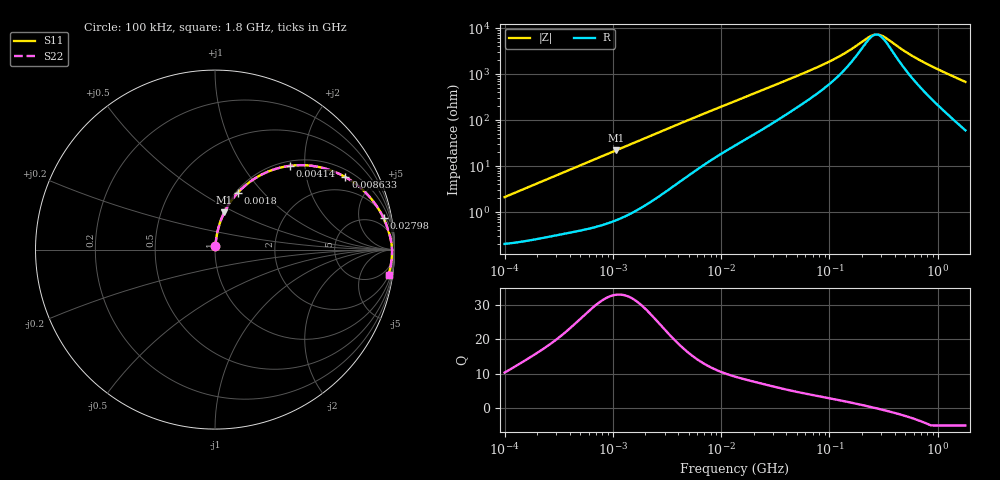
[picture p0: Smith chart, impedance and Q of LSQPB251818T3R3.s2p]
! LSQPB251818T3R3  S-PARAMETER MODEL  ( General Type )
! Model Generated by TAIYO YUDEN Corporation (http://www.ty-top.com)
! Version 2.0
! TAIYO YUDEN Control No. 100810NG19SB-FKC
! Copyright(c) 2009 TAIYO YUDEN CO.,LTD. All Rights Reserved.
! Product Description (link to TY-COMPAS)
! https://ds.yuden.co.jp/TYCOMPAS/or/detail?pn=LSQPB251818T3R3M&u=M
! Products Name : Inductors
! Characteristics :
!  Inductance : 3.3 uH , SRF(min) : 150 MHz , DC Resistance(max) : 0.2275 Ohm
!  Rated Current : Saturation :1450 mA , Temp Rise : 860 mA (40 degC)
!  Case Size : 2.5 x 1.8 / 0.098 x 0.071 [mm/inch] , Thickness : 1.8 / 0.071 [mm/inch]
!  (Conditions: Temperature = 25 degC , DC Bias Current/Voltage = 0A / 0V)
! External Node Assignments :
!  1  o---GGG---o  2
! GND o---------o GND
! Frequency Range : 0.1MHz  -  1800MHz  [ 402 STEP ]
# MHz S RI R 50
! Freq[MHz].  S11 Real  S11 Imag  S21 Real  S21 Imag  S12 Real  S12 Imag  S22 Real  S22 Imag
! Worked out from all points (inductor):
!   401 points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, 100 kHz to 1.8 GHz, reference 50 ohm
!   read as one part in series: L = 3.35 uH near 105 kHz
!   highest Q = 33 at 1.076 MHz (marker M1), where L = 3.26 uH
!   self-resonance near 270.2 MHz
!   S11 on the Smith chart (normalised r, x): 100 kHz: 1.00, +0.04; 1.8 MHz: 1.02, +0.74; 4.14 MHz: 1.09, +1.67; 8.633 MHz: 1.30, +3.39; 27.98 MHz: 3, +10; 1.8 GHz: 2, -13
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0.1  0.00248 0.021  0.9975 -0.021  0.9975 -0.021  0.00248 0.021
0.253659  0.00565 0.0524  0.9943 -0.0524  0.9943 -0.0524  0.00565 0.0524
0.516129  0.0151 0.1044  0.9849 -0.1044  0.9849 -0.1044  0.0151 0.1044
1.076226  0.0521 0.2076  0.9479 -0.2076  0.9479 -0.2076  0.0521 0.2076
1.800136  0.1272 0.3171  0.8728 -0.3171  0.8728 -0.3171  0.1272 0.3171
2.66389  0.2365 0.4052  0.7635 -0.4052  0.7635 -0.4052  0.2365 0.4052
4.140031  0.4168 0.4666  0.5832 -0.4666  0.5832 -0.4666  0.4168 0.4666
5.833619  0.5726 0.4614  0.4274 -0.4614  0.4274 -0.4614  0.5726 0.4614
8.632747  0.7262 0.4042  0.2738 -0.4042  0.2738 -0.4042  0.7262 0.4042
13.41641  0.8447 0.3119  0.1553 -0.3119  0.1553 -0.3119  0.8447 0.3119
18.90474  0.9014 0.2417  0.0986 -0.2417  0.0986 -0.2417  0.9014 0.2417
27.97575  0.9397 0.1739  0.0603 -0.1739  0.0603 -0.1739  0.9397 0.1739
69.24595  0.9749 0.0736  0.0251 -0.0736  0.0251 -0.0736  0.9749 0.0736
127.7465  0.983 0.0348  0.017 -0.0348  0.017 -0.0348  0.983 0.0348
247.5026  0.9862 0.00383  0.0138 -0.00383  0.0138 -0.00383  0.9862 0.00383
272.9811  0.9864 -0.000441  0.0136 0.000441  0.0136 0.000441  0.9864 -0.000441
293.7968  0.9865 -0.00365  0.0135 0.00365  0.0135 0.00365  0.9865 -0.00365
357.3983  0.9866 -0.0124  0.0134 0.0124  0.0134 0.0124  0.9866 -0.0124
503.6016  0.9861 -0.0291  0.0139 0.0291  0.0139 0.0291  0.9861 -0.0291
692.4421  0.9847 -0.0476  0.0153 0.0476  0.0153 0.0476  0.9847 -0.0476
1102.831  0.98 -0.0837  0.02 0.0837  0.02 0.0837  0.98 -0.0837
1800  0.9668 -0.1403  0.0332 0.1403  0.0332 0.1403  0.9668 -0.1403
